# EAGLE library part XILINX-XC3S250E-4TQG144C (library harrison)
Xilinx FPGA
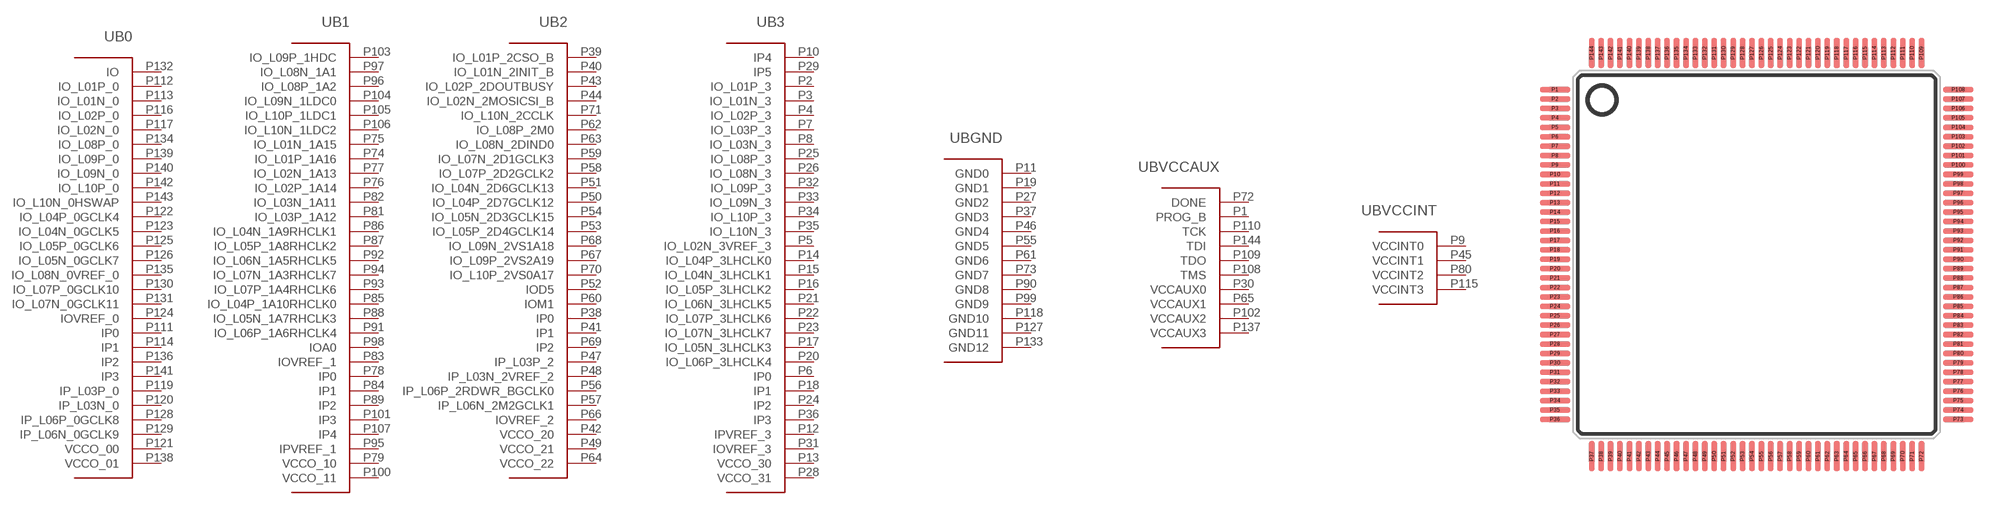
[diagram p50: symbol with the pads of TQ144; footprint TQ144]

Designator prefix U; gates B0=XC3S250ETQ144_0 B1=XC3S250ETQ144_1 B2=XC3S250ETQ144_2 B3=XC3S250ETQ144_3 BGND=XC3S250ETQ144_GND BVCCAUX=XC3S250ETQ144_VCCAUX BVCCINT=XC3S250ETQ144_VCCINT

## XILINX-XC3S250E-4TQG144C (RNUMBER: R00701; VAL: XC3S100E-4TQG144C)  [TQ144]
P1  BVCCAUX:PROG_B
P2  B3:IO_L01P_3
P3  B3:IO_L01N_3
P4  B3:IO_L02P_3
P5  B3:IO_L02N_3VREF_3
P6  B3:IP0  in
P7  B3:IO_L03P_3
P8  B3:IO_L03N_3
P9  BVCCINT:VCCINT0  pwr
P10  B3:IP4  in
P11  BGND:GND0  pwr
P12  B3:IPVREF_3  in
P13  B3:VCCO_30  pwr
P14  B3:IO_L04P_3LHCLK0
P15  B3:IO_L04N_3LHCLK1
P16  B3:IO_L05P_3LHCLK2
P17  B3:IO_L05N_3LHCLK3
P18  B3:IP1  in
P19  BGND:GND1  pwr
P20  B3:IO_L06P_3LHCLK4
P21  B3:IO_L06N_3LHCLK5
P22  B3:IO_L07P_3LHCLK6
P23  B3:IO_L07N_3LHCLK7
P24  B3:IP2  in
P25  B3:IO_L08P_3
P26  B3:IO_L08N_3
P27  BGND:GND2  pwr
P28  B3:VCCO_31  pwr
P29  B3:IP5  in
P30  BVCCAUX:VCCAUX0  pwr
P31  B3:IOVREF_3
P32  B3:IO_L09P_3
P33  B3:IO_L09N_3
P34  B3:IO_L10P_3
P35  B3:IO_L10N_3
P36  B3:IP3  in
P37  BGND:GND3  pwr
P38  B2:IP0  in
P39  B2:IO_L01P_2CSO_B
P40  B2:IO_L01N_2INIT_B
P41  B2:IP1  in
P42  B2:VCCO_20  pwr
P43  B2:IO_L02P_2DOUTBUSY
P44  B2:IO_L02N_2MOSICSI_B
P45  BVCCINT:VCCINT1  pwr
P46  BGND:GND4  pwr
P47  B2:IP_L03P_2  in
P48  B2:IP_L03N_2VREF_2  in
P49  B2:VCCO_21  pwr
P50  B2:IO_L04P_2D7GCLK12
P51  B2:IO_L04N_2D6GCLK13
P52  B2:IOD5
P53  B2:IO_L05P_2D4GCLK14
P54  B2:IO_L05N_2D3GCLK15
P55  BGND:GND5  pwr
P56  B2:IP_L06P_2RDWR_BGCLK0  in
P57  B2:IP_L06N_2M2GCLK1  in
P58  B2:IO_L07P_2D2GCLK2
P59  B2:IO_L07N_2D1GCLK3
P60  B2:IOM1
P61  BGND:GND6  pwr
P62  B2:IO_L08P_2M0
P63  B2:IO_L08N_2DIND0
P64  B2:VCCO_22  pwr
P65  BVCCAUX:VCCAUX1  pwr
P66  B2:IOVREF_2
P67  B2:IO_L09P_2VS2A19
P68  B2:IO_L09N_2VS1A18
P69  B2:IP2  in
P70  B2:IO_L10P_2VS0A17
P71  B2:IO_L10N_2CCLK
P72  BVCCAUX:DONE
P73  BGND:GND7  pwr
P74  B1:IO_L01P_1A16
P75  B1:IO_L01N_1A15
P76  B1:IO_L02P_1A14
P77  B1:IO_L02N_1A13
P78  B1:IP0  in
P79  B1:VCCO_10  pwr
P80  BVCCINT:VCCINT2  pwr
P81  B1:IO_L03P_1A12
P82  B1:IO_L03N_1A11
P83  B1:IOVREF_1
P84  B1:IP1  in
P85  B1:IO_L04P_1A10RHCLK0
P86  B1:IO_L04N_1A9RHCLK1
P87  B1:IO_L05P_1A8RHCLK2
P88  B1:IO_L05N_1A7RHCLK3
P89  B1:IP2  in
P90  BGND:GND8  pwr
P91  B1:IO_L06P_1A6RHCLK4
P92  B1:IO_L06N_1A5RHCLK5
P93  B1:IO_L07P_1A4RHCLK6
P94  B1:IO_L07N_1A3RHCLK7
P95  B1:IPVREF_1  in
P96  B1:IO_L08P_1A2
P97  B1:IO_L08N_1A1
P98  B1:IOA0
P99  BGND:GND9  pwr
P100  B1:VCCO_11  pwr
P101  B1:IP3  in
P102  BVCCAUX:VCCAUX2  pwr
P103  B1:IO_L09P_1HDC
P104  B1:IO_L09N_1LDC0
P105  B1:IO_L10P_1LDC1
P106  B1:IO_L10N_1LDC2
P107  B1:IP4  in
P108  BVCCAUX:TMS
P109  BVCCAUX:TDO
P110  BVCCAUX:TCK
P111  B0:IP0  in
P112  B0:IO_L01P_0
P113  B0:IO_L01N_0
P114  B0:IP1  in
P115  BVCCINT:VCCINT3  pwr
P116  B0:IO_L02P_0
P117  B0:IO_L02N_0
P118  BGND:GND10  pwr
P119  B0:IP_L03P_0  in
P120  B0:IP_L03N_0  in
P121  B0:VCCO_00  pwr
P122  B0:IO_L04P_0GCLK4
P123  B0:IO_L04N_0GCLK5
P124  B0:IOVREF_0
P125  B0:IO_L05P_0GCLK6
P126  B0:IO_L05N_0GCLK7
P127  BGND:GND11  pwr
P128  B0:IP_L06P_0GCLK8  in
P129  B0:IP_L06N_0GCLK9  in
P130  B0:IO_L07P_0GCLK10
P131  B0:IO_L07N_0GCLK11
P132  B0:IO
P133  BGND:GND12  pwr
P134  B0:IO_L08P_0
P135  B0:IO_L08N_0VREF_0
P136  B0:IP2  in
P137  BVCCAUX:VCCAUX3  pwr
P138  B0:VCCO_01  pwr
P139  B0:IO_L09P_0
P140  B0:IO_L09N_0
P141  B0:IP3  in
P142  B0:IO_L10P_0
P143  B0:IO_L10N_0HSWAP
P144  BVCCAUX:TDI

## Footprint TQ144 (pad centres in mm)
smd 1.6 x 0.3: P1 -10.7,8.75; P2 -10.7,8.25; P3 -10.7,7.75; P4 -10.7,7.25; P5 -10.7,6.75; P6 -10.7,6.25; P7 -10.7,5.75; P8 -10.7,5.25; P9 -10.7,4.75; P10 -10.7,4.25; P11 -10.7,3.75; P12 -10.7,3.25; P13 -10.7,2.75; P14 -10.7,2.25; P15 -10.7,1.75; P16 -10.7,1.25; P17 -10.7,0.75; P18 -10.7,0.25; P19 -10.7,-0.25; P20 -10.7,-0.75; P21 -10.7,-1.25; P22 -10.7,-1.75; P23 -10.7,-2.25; P24 -10.7,-2.75; P25 -10.7,-3.25; P26 -10.7,-3.75; P27 -10.7,-4.25; P28 -10.7,-4.75; P29 -10.7,-5.25; P30 -10.7,-5.75; P31 -10.7,-6.25; P32 -10.7,-6.75; P33 -10.7,-7.25; P34 -10.7,-7.75; P35 -10.7,-8.25; P36 -10.7,-8.75; P73 10.7,-8.75; P74 10.7,-8.25; P75 10.7,-7.75; P76 10.7,-7.25; P77 10.7,-6.75; P78 10.7,-6.25; P79 10.7,-5.75; P80 10.7,-5.25; P81 10.7,-4.75; P82 10.7,-4.25; P83 10.7,-3.75; P84 10.7,-3.25; P85 10.7,-2.75; P86 10.7,-2.25; P87 10.7,-1.75; P88 10.7,-1.25; P89 10.7,-0.75; P90 10.7,-0.25; P91 10.7,0.25; P92 10.7,0.75; P93 10.7,1.25; P94 10.7,1.75; P95 10.7,2.25; P96 10.7,2.75; P97 10.7,3.25; P98 10.7,3.75; P99 10.7,4.25; P100 10.7,4.75; P101 10.7,5.25; P102 10.7,5.75; P103 10.7,6.25; P104 10.7,6.75; P105 10.7,7.25; P106 10.7,7.75; P107 10.7,8.25; P108 10.7,8.75
smd 0.3 x 1.6: P37 -8.75,-10.7; P38 -8.25,-10.7; P39 -7.75,-10.7; P40 -7.25,-10.7; P41 -6.75,-10.7; P42 -6.25,-10.7; P43 -5.75,-10.7; P44 -5.25,-10.7; P45 -4.75,-10.7; P46 -4.25,-10.7; P47 -3.75,-10.7; P48 -3.25,-10.7; P49 -2.75,-10.7; P50 -2.25,-10.7; P51 -1.75,-10.7; P52 -1.25,-10.7; P53 -0.75,-10.7; P54 -0.25,-10.7; P55 0.25,-10.7; P56 0.75,-10.7; P57 1.25,-10.7; P58 1.75,-10.7; P59 2.25,-10.7; P60 2.75,-10.7; P61 3.25,-10.7; P62 3.75,-10.7; P63 4.25,-10.7; P64 4.75,-10.7; P65 5.25,-10.7; P66 5.75,-10.7; P67 6.25,-10.7; P68 6.75,-10.7; P69 7.25,-10.7; P70 7.75,-10.7; P71 8.25,-10.7; P72 8.75,-10.7; P109 8.75,10.7; P110 8.25,10.7; P111 7.75,10.7; P112 7.25,10.7; P113 6.75,10.7; P114 6.25,10.7; P115 5.75,10.7; P116 5.25,10.7; P117 4.75,10.7; P118 4.25,10.7; P119 3.75,10.7; P120 3.25,10.7; P121 2.75,10.7; P122 2.25,10.7; P123 1.75,10.7; P124 1.25,10.7; P125 0.75,10.7; P126 0.25,10.7; P127 -0.25,10.7; P128 -0.75,10.7; P129 -1.25,10.7; P130 -1.75,10.7; P131 -2.25,10.7; P132 -2.75,10.7; P133 -3.25,10.7; P134 -3.75,10.7; P135 -4.25,10.7; P136 -4.75,10.7; P137 -5.25,10.7; P138 -5.75,10.7; P139 -6.25,10.7; P140 -6.75,10.7; P141 -7.25,10.7; P142 -7.75,10.7; P143 -8.25,10.7; P144 -8.75,10.7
